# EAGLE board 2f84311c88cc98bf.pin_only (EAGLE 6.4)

Size 31.75 x 44.45 mm. Coordinates in mm from the lower left corner, seen from the top.
Outline: 31.75,41.91 31.75,2.54 arc-90 29.21,0 2.54,0 arc-90 0,2.54 0,9.27 1.14,9.27 1.14,13.08 0,13.08 0,41.91 arc-90 2.54,44.45 29.21,44.45 arc-90 31.75,41.91
Copper layers (1*16): Top 0.035mm / dielectric 1.5mm / Bottom 0.035mm
Design rules "adafruit *": minimum track width 6mil, minimum drill 15.5mil, track to track 8mil, track to pad 6mil, pad to pad 8mil, via to via 8mil, smd to smd 8mil, copper to edge 10mil, drill to drill 8mil, minimum pad ring 10mil, minimum via ring 8mil, stop-mask expansion 2mil, vias tented up to drill 20mil, thermal gap 10mil
tRestrict: area 16.1,22.4 to 16.3,29.2; area 19.8,31.5 to 20.3,31.8; area 22.7,31.5 to 23.1,31.8; area 16.3,22.2 to 24.5,22.4; area 26.8,22.5 to 27.2,30.5; area 17.5,31.5 to 18,31.8; area 16,30.2 to 16.3,30.7

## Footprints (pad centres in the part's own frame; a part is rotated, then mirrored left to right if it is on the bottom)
1X01-CLEANBIG = drill 1.016 pad 1.778: 1 0,0
0805-NO = smd 1.3 x 1.5: 1 -0.95,0; 2 0.95,0
C1210 = smd 1.6 x 2.7: 1 -1.4,0; 2 1.4,0
RESPACK_4X0603 = smd 0.45 x 0.9: 1 -1.3,-0.85; 2 -0.4,-0.85; 3 0.4,-0.85; 4 1.3,-0.85; 5 1.3,0.85; 6 0.4,0.85; 7 -0.4,0.85; 8 -1.3,0.85
CHIPLED_0805_NOOUTLINE = smd 1.2 x 1.2: A 0,-1.05; C 0,1.05
JSTPH2 = smd 1 x 4.6: 1 -1,-3.7; 2 1,-3.7 | smd 1.6 x 3.4: NC1 -3.4,1.5; NC2 3.4,1.5
SOD-123 = smd 1.4 x 1.4: A 1.85,0; C -1.85,0
SOT363 = smd 0.5 x 0.5: 1 -0.75,-0.9; 3 0.75,-0.9; 4 0.75,0.9; 6 -0.75,0.9 | smd 0.4 x 0.5: 2 0,-0.9; 5 0,0.9
SOD-323 = smd 1.35 x 0.8: A 1.27,0; C -1.27,0
FIDUCIAL_1MM = smd 1 x 1: 1 0,0
TSSOP14 = smd 0.35 x 0.9: 1 -1.95,-2.925; 2 -1.3,-2.925; 3 -0.65,-2.925; 4 0,-2.925; 5 0.65,-2.925; 6 1.3,-2.925; 7 1.95,-2.925; 8 1.95,2.925; 9 1.3,2.925; 10 0.65,2.925; 11 0,2.925; 12 -0.65,2.925; 13 -1.3,2.925; 14 -1.95,2.925
1X12-CB = drill 1.016 pad 1.778: 1 -13.97,0; 2 -11.43,0; 3 -8.89,0; 4 -6.35,0; 5 -3.81,0; 6 -1.27,0; 7 1.27,0; 8 3.81,0; 9 6.35,0; 10 8.89,0; 11 11.43,0; 12 13.97,0
1X02_ROUND = drill 1 pad 1.778: 1 -1.27,0; 2 1.27,0
SC59-BEC = smd 1 x 1.4: B -0.95,-1.2; C 0,1.2; E 0.95,-1.2
BTN_KMR2_4.6X2.8 = smd 0.9 x 1: A 2.05,0.8; A' -2.05,0.8; B 2.05,-0.8; B' -2.05,-0.8
TP11R = smd 1.1 x 1.1: TP 0,0
SIM800L = smd 1.1 x 0.9: 1 -8.1,5.6; 2 -8.1,4.2; 3 -8.1,2.8; 4 -8.1,1.4; 5 -8.1,0; 6 -8.1,-1.4; 7 -8.1,-2.8; 8 -8.1,-4.2; 9 -8.1,-5.6; 22 8.1,-5.6; 23 8.1,-4.2; 24 8.1,-2.8; 25 8.1,-1.4; 26 8.1,0; 27 8.1,1.4; 28 8.1,2.8; 29 8.1,4.2; 30 8.1,5.6; 43 -6.36,5.6; 44 -6.36,4.2; 45 -6.36,2.8; 46 -6.36,1.4; 47 -6.36,0; 48 -6.36,-1.4; 49 -6.36,-2.8; 50 -6.36,-4.2; 51 -6.36,-5.6; 60 6.36,-5.6; 61 6.36,-4.2; 62 6.36,-2.8; 63 6.36,-1.4; 64 6.36,0; 65 6.36,1.4; 66 6.36,2.8; 67 6.36,4.2; 68 6.36,5.6 | smd 0.9 x 1.1: 10 -7.7,-7.1; 11 -6.3,-7.1; 12 -4.9,-7.1; 13 -3.5,-7.1; 14 -2.1,-7.1; 15 -0.7,-7.1; 16 0.7,-7.1; 17 2.1,-7.1; 18 3.5,-7.1; 19 4.9,-7.1; 20 6.3,-7.1; 21 7.7,-7.1; 31 7.7,7.1; 32 6.3,7.1; 33 4.9,7.1; 34 3.5,7.1; 35 2.1,7.1; 36 0.7,7.1; 37 -0.7,7.1; 38 -2.1,7.1; 39 -3.5,7.1; 40 -4.9,7.1; 41 -6.3,7.1; 42 -7.7,7.1; 52 -4.9,-5.5; 53 -3.5,-5.5; 54 -2.1,-5.5; 55 -0.7,-5.5; 56 0.7,-5.5; 57 2.1,-5.5; 58 3.5,-5.5; 59 4.9,-5.5; 69 4.9,5.5; 70 3.5,5.5; 71 2.1,5.5; 72 0.7,5.5; 73 -0.7,5.5; 74 -2.1,5.5; 75 -3.5,5.5; 76 -4.9,5.5 | smd 1.5 x 1.5: 77 -3.9,3 | smd 2.3 x 2.7: 78 -3.9,0; 79 -3.9,-3; 80 -1.3,-3; 81 1.3,-3; 82 3.9,-3; 83 3.9,0; 84 3.9,3; 85 1.3,3; 86 -1.3,3; 87 -1.3,0; 88 1.3,0
SOT23-5 = smd 0.55 x 1.2: 1 -0.95,-1.3; 2 0,-1.3; 3 0.95,-1.3; 4 0.95,1.3; 5 -0.95,1.3
MOUNTINGHOLE_2.5_PLATED = drill 2.5 pad 3.2: P$1 0,0
SMA_EDGELAUNCH_UFL = smd 4.064 x 1.524: GND@1 2.032,-2.54; GND@2 2.032,2.54 | smd 4.064 x 1.524 bottom: GND@3 2.032,2.54; GND@4 2.032,-2.54 | smd 2.032 x 1.016: P 3.048,0
4UCONN_20329 = smd 1 x 2: BASE@1 -0.75,-2; BASE@2 0.75,-2 | smd 0.4 x 1.35: D+ 0,0.775; D- -0.65,0.775; GND 1.3,0.775; ID 0.65,0.775; VBUS -1.3,0.775 | drill 0.7 offset: SPRT@1 -3.3,0.9; SPRT@2 3.3,0.9 | drill 0.6 pad 2.5 square: SPRT@3 -3.6,-1.9; SPRT@4 3.6,-1.9 | hole 0.7: -1.95,0; 1.95,0
4UCONN_18510 = smd 1.5 x 2.5: 1-GND 2.8,-3.3; 2-TIP 9.3,3.4; 3-OUTER_SLEEVE 5.5,-3.3 | smd 1.5 x 3.4: 4-INNER_SLEEVE 2.8,2.9 | hole 1.3: 10.5,0
C707_10M006_512_2 = smd 1.7 x 1.3: C1 -12.85,-3.915; C2 -12.85,-1.375; C3 -12.85,1.165; C5 12.85,-3.915; C6 12.85,-1.375; C7 12.85,1.165

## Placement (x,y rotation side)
ADC  [1X01-CLEANBIG]  11.18,20.32 0 top
C1  10µF  [0805-NO]  8.13,21.08 0 top
C2  33pF  [0805-NO]  2.03,5.21 180 top
C3  10pF  [0805-NO]  5.59,5.21 0 top
C4  33pF  [0805-NO]  12.06,15.62 180 top
C5  10pF  [0805-NO]  13.32,36.94 90 top
C6  33pF  [0805-NO]  9.99,38.31 0 top
C7  100uF  [C1210]  9.78,29.34 270 top
C9  10uF  [0805-NO]  26.92,16.76 270 top
C10  10pF  [0805-NO]  11.94,17.4 180 top
C11  10uF  [0805-NO]  5.97,15.75 0 top
C14  33pF  [RESPACK_4X0603]  19.56,9.78 0 top
C15  10pF  [RESPACK_4X0603]  19.56,13.34 180 top
C16  33pF  [RESPACK_4X0603]  14.86,13.34 0 top
C17  10pF  [RESPACK_4X0603]  14.86,9.53 0 top
CHRG  ORANGE  [CHIPLED_0805_NOOUTLINE]  2.16,28.08 270 top
CN2  JSTPH  [JSTPH2]  3.56,35.05 90 top
D1  MMSZ5231BT1G  [SOD-123]  10.67,34.54 270 top
D2  SMF05C  [SOT363]  21.21,17.02 90 top
D3  1N4148  [SOD-323]  25.91,41.91 270 top
D4  1N4148  [SOD-323]  28.19,5.46 0 top
D5  1N4148  [SOD-323]  24.51,6.99 90 top
D6  1N4148  [SOD-323]  28.19,7.11 0 top
DONE  GREEN  [CHIPLED_0805_NOOUTLINE]  2.17,29.93 90 top
FID1  FIDUCIAL""  [FIDUCIAL_1MM]  5.97,11.81 0 top
FID2  FIDUCIAL""  [FIDUCIAL_1MM]  2.03,35.81 0 top
FID3  FIDUCIAL""  [FIDUCIAL_1MM]  25.91,11.94 0 top
FID4  FIDUCIAL""  [FIDUCIAL_1MM]  28.45,39.12 0 bottom
FID5  FIDUCIAL""  [FIDUCIAL_1MM]  3.17,3.56 0 bottom
IC1  74VHCT125PW  [TSSOP14]  26.54,11.94 270 top
JP1  [1X12-CB]  16,1.52 180 top
JP2  MIC  [1X02_ROUND]  18.54,5.21 0 top
JP3  BUZZ  [1X02_ROUND]  23.75,41.91 90 top
NETSTAT  BLUE  [CHIPLED_0805_NOOUTLINE]  21.34,36.96 0 top
PWM  [1X01-CLEANBIG]  30.48,38.61 0 top
PWRSTAT  GREEN  [CHIPLED_0805_NOOUTLINE]  12.7,6.48 270 top
Q1  DTC143ZUAT106  [SC59-BEC]  26.67,37.47 270 top
R1  470  [0805-NO]  5.71,28.19 0 top
R2  1K  [0805-NO]  5.73,29.97 0 top
R3  2K  [0805-NO]  11.05,23.11 90 top
R4  1K  [0805-NO]  12.57,4.83 0 top
R5  1K  [0805-NO]  23.37,36.96 90 top
SW1  KMR2  [BTN_KMR2_4.6X2.8]  7.49,42.42 0 top
TP1  TPTP11R  [TP11R]  29.59,17.27 0 top
U1  SIM800H/L  [SIM800L]  21.59,26.96 0 top
U2  MCP73831T-2ACI/OT  [SOT23-5]  8.13,24.64 180 top
U$10  [ADAFRUIT_5MM]  14.48,35.18 0 top
U$26  [FONA_LOGO]  4.95,23.11 90 bottom
U$33  MOUNTINGHOLE2.5  [MOUNTINGHOLE_2.5_PLATED]  29.21,41.91 90 top
U$34  MOUNTINGHOLE2.5  [MOUNTINGHOLE_2.5_PLATED]  2.54,41.91 90 top
U$36  [ADAFRUIT_5MM]  18.92,36.32 0 bottom
VBUS  [1X01-CLEANBIG]  7.49,18.03 0 top
X1  [SMA_EDGELAUNCH_UFL]  16.76,44.2 270 top
X2  MicroB  [4UCONN_20329]  4.32,22.1 270 top
X4  [4UCONN_18510]  0,11.18 0 top
X6  SIM_LOCKAMPHENOL  [C707_10M006_512_2]  22.48,22.86 270 bottom

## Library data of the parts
ADC PWM VBUS = adafruit
C1-C6 C9-C11 C14-C17 CHRG CN2 D1-D3 DONE JP2 JP3 NETSTAT PWRSTAT R1-R5 SW1 U1 U2 U$10 U$26 U$36 X1 X2 X4 = microbuilder
C7 = rcl
D4-D6 = microbuilder; COMPANY: ADAFRUIT INDUSTRIES; DRAWN: KTOWN; REV: A
FID1-FID5 U$33 U$34 = microbuilder; BOM: EXCLUDE
IC1 = 74xx-us
JP1 = adafruit2
Q1 = transistor
TP1 = testpad
X6 = microbuilder; OC_FARNELL: unknown; OC_NEWARK: unknown

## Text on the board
tPlace: Key | PWM | Net | 5V | ADC | 2.8V | Mic | PWR | + | - | Bat | GND | Key | + | SPKR | Rst | PS | RI | TX | RX | NS | Vio | -
bPlace: Buzzer | + | - | adafruit! | 3.7V LiPoly / 0.5A charge | USB Charging | Only | FONA MiniGSM | Cell-phone / Data/SMS | 2G GSM / SIM Card | TRRS: / LR-M | Vio: I/O Level 3-5VDC

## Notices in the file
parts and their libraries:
microbuilder: This work is placed in the public domain, and may be freely used for commercial and non-commercial work with the following conditions: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
